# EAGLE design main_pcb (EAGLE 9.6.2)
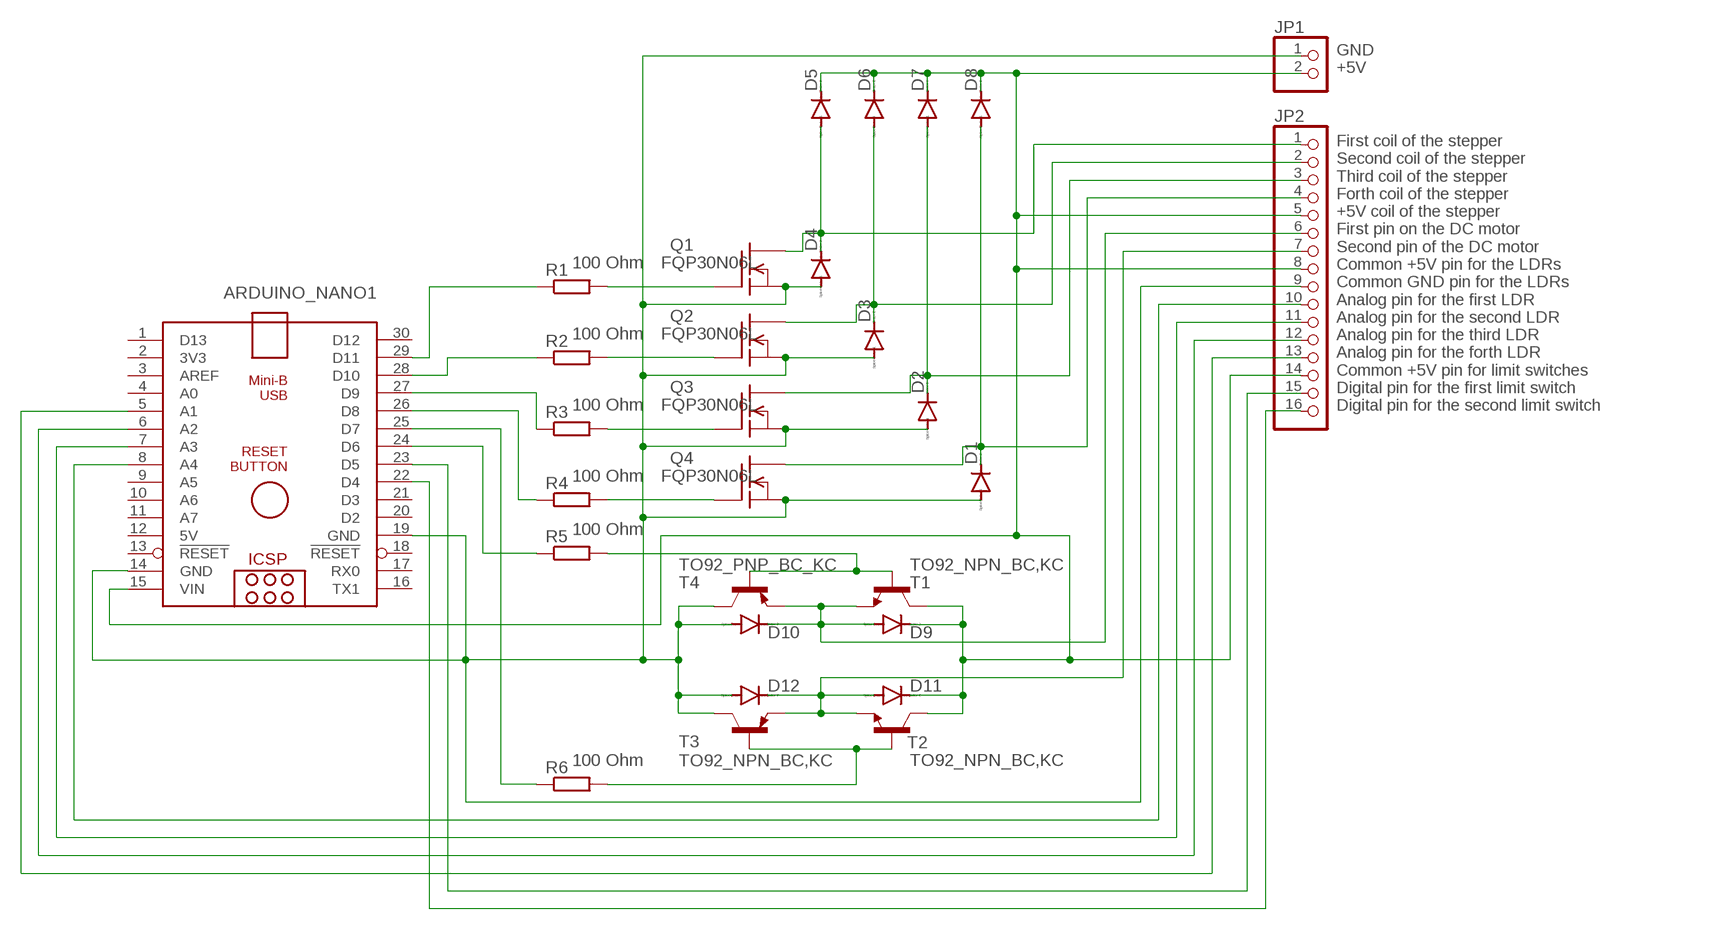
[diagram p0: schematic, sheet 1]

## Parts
ARDUINO_NANO1  ARDUINO_NANO  [ARDUINO_NANO]
D1  DIODY_1N,KADO35-7  [DO35-7]
D2  DIODY_1N,KADO35-7  [DO35-7]
D3  DIODY_1N,KADO35-7  [DO35-7]
D4  DIODY_1N,KADO35-7  [DO35-7]
D5  DIODY_1N,KADO35-7  [DO35-7]
D6  DIODY_1N,KADO35-7  [DO35-7]
D7  DIODY_1N,KADO35-7  [DO35-7]
D8  DIODY_1N,KADO35-7  [DO35-7]
D9  DIODY_1N,KADO35-7  [DO35-7]
D10  DIODY_1N,KADO35-7  [DO35-7]
D11  DIODY_1N,KADO35-7  [DO35-7]
D12  DIODY_1N,KADO35-7  [DO35-7]
JP1  PINHD-1X2  [1X02]
JP2  PINHD-1X16  [1X16]
Q1  BUZ10  [TO220]
Q2  BUZ10  [TO220]
Q3  BUZ10  [TO220]
Q4  BUZ10  [TO220]
R1  R-EU_0204/7  [0204/7]
R2  R-EU_0204/7  [0204/7]
R3  R-EU_0204/7  [0204/7]
R4  R-EU_0204/7  [0204/7]
R5  R-EU_0204/7  [0204/7]
R6  R-EU_0204/7  [0204/7]
T1  TO92_NPN_BC,KC  [TO92]
T2  TO92_NPN_BC,KC  [TO92]
T3  TO92_PNP_BC_KC  [TO92]
T4  TO92_PNP_BC_KC  [TO92]

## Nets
+5V: ARDUINO_NANO1.15(VIN) D5.C D6.C D7.C D8.C D9.C D11.C JP1.2 JP2.5 JP2.8 JP2.14 T1.3(C) T2.3(C)
GND: ARDUINO_NANO1.14(GND) ARDUINO_NANO1.19(GND) D1.A D2.A D3.A D4.A D10.A D12.A JP1.1 JP2.9 Q1.3(S) Q2.3(S) Q3.3(S) Q4.3(S) T3.3(C) T4.3(C)
N$1: ARDUINO_NANO1.29(D11) R1.1
N$2: ARDUINO_NANO1.28(D10) R2.1
N$3: ARDUINO_NANO1.27(D9) R3.1
N$4: ARDUINO_NANO1.26(D8) R4.1
N$5: Q1.1(G) R1.2
N$6: Q2.1(G) R2.2
N$7: Q3.1(G) R3.2
N$8: Q4.1(G) R4.2
N$9: D9.A D10.C JP2.6 T1.1(E) T4.1(E)
N$10: ARDUINO_NANO1.23(D5) JP2.15
N$11: ARDUINO_NANO1.22(D4) JP2.16
N$13: D11.A D12.C JP2.7 T2.1(E) T3.1(E)
N$14: D2.C D7.A JP2.3 Q3.2(D)
N$15: D3.C D6.A JP2.2 Q2.2(D)
N$16: D4.C D5.A JP2.1 Q1.2(D)
N$17: R5.2 T1.2(B) T4.2(B)
N$18: D1.C D8.A JP2.4 Q4.2(D)
N$19: R6.2 T2.2(B) T3.2(B)
N$20: ARDUINO_NANO1.25(D7) R6.1
N$21: ARDUINO_NANO1.24(D6) R5.1
N$23: ARDUINO_NANO1.8(A4) JP2.10
N$25: ARDUINO_NANO1.7(A3) JP2.11
N$26: ARDUINO_NANO1.6(A2) JP2.12
N$27: ARDUINO_NANO1.5(A1) JP2.13
Unconnected: ARDUINO_NANO1.1(D13) ARDUINO_NANO1.2(3V3) ARDUINO_NANO1.3(AREF) ARDUINO_NANO1.4(A0) ARDUINO_NANO1.9(A5) ARDUINO_NANO1.10(A6) ARDUINO_NANO1.11(A7) ARDUINO_NANO1.13(!RESET) ARDUINO_NANO1.16(TX1) ARDUINO_NANO1.17(RX0) ARDUINO_NANO1.18(!RESET) ARDUINO_NANO1.20(D2) ARDUINO_NANO1.21(D3) ARDUINO_NANO1.30(D12)

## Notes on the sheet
- GND
  +5V
- 100 Ohm | FQP30N06L
- 100 Ohm | FQP30N06L
- 100 Ohm | FQP30N06L
- First coil of the stepper
  Second coil of the stepper
  Third coil of the stepper
  Forth coil of the stepper
  +5V coil of the stepper
  First pin on the DC motor
  Second pin of the DC motor
  Common +5V pin for the LDRs
  Common GND pin for the LDRs
  Analog pin for the first LDR
  Analog pin for the second LDR
  Analog pin for the third LDR
  Analog pin for the forth LDR
  Common +5V pin for limit switches
  Digital pin for the first limit switch
  Digital pin for the second limit switch
- 100 Ohm | FQP30N06L
- 100 Ohm
- T4
- 100 Ohm
- T3
  TO92_NPN_BC,KC
- TO92_NPN_BC,KC

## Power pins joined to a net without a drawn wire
5V: ARDUINO_NANO1.12(5V)

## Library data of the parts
ARDUINO_NANO1 = ArduinoNanoV30:ARDUINO_NANO: Arduino Nano V3.0 Overview: The Arduino Nano is a small, complete, and breadboard-friendly board based on the ATmega328 (Arduino Nano 3.x) or ATmega168 (Arduino Nano 2.x). It has more or less the same functionality of the Arduino Duemilanove, but in a different package. It lacks only a DC power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
D1-D12 = knihovna praxe 123:DIODY_1N,KA: DIODE
JP1 = pinhead:PINHD-1X2: PIN HEADER
JP2 = pinhead:PINHD-1X16: PIN HEADER
Q1-Q4 = transistor-fet:BUZ10: N-Channel Enhancement MOSFET 50V; 20A; 0,080Ohm
R1-R6 = rcl:R-EU_: RESISTOR, European symbol; SPICEPREFIX: R
T1 T2 = knihovna praxe 123:TO92_NPN_BC,KC: NPN TRANSISTOR
T3 T4 = knihovna praxe 123:TO92_PNP_BC_KC: PNP Transistor

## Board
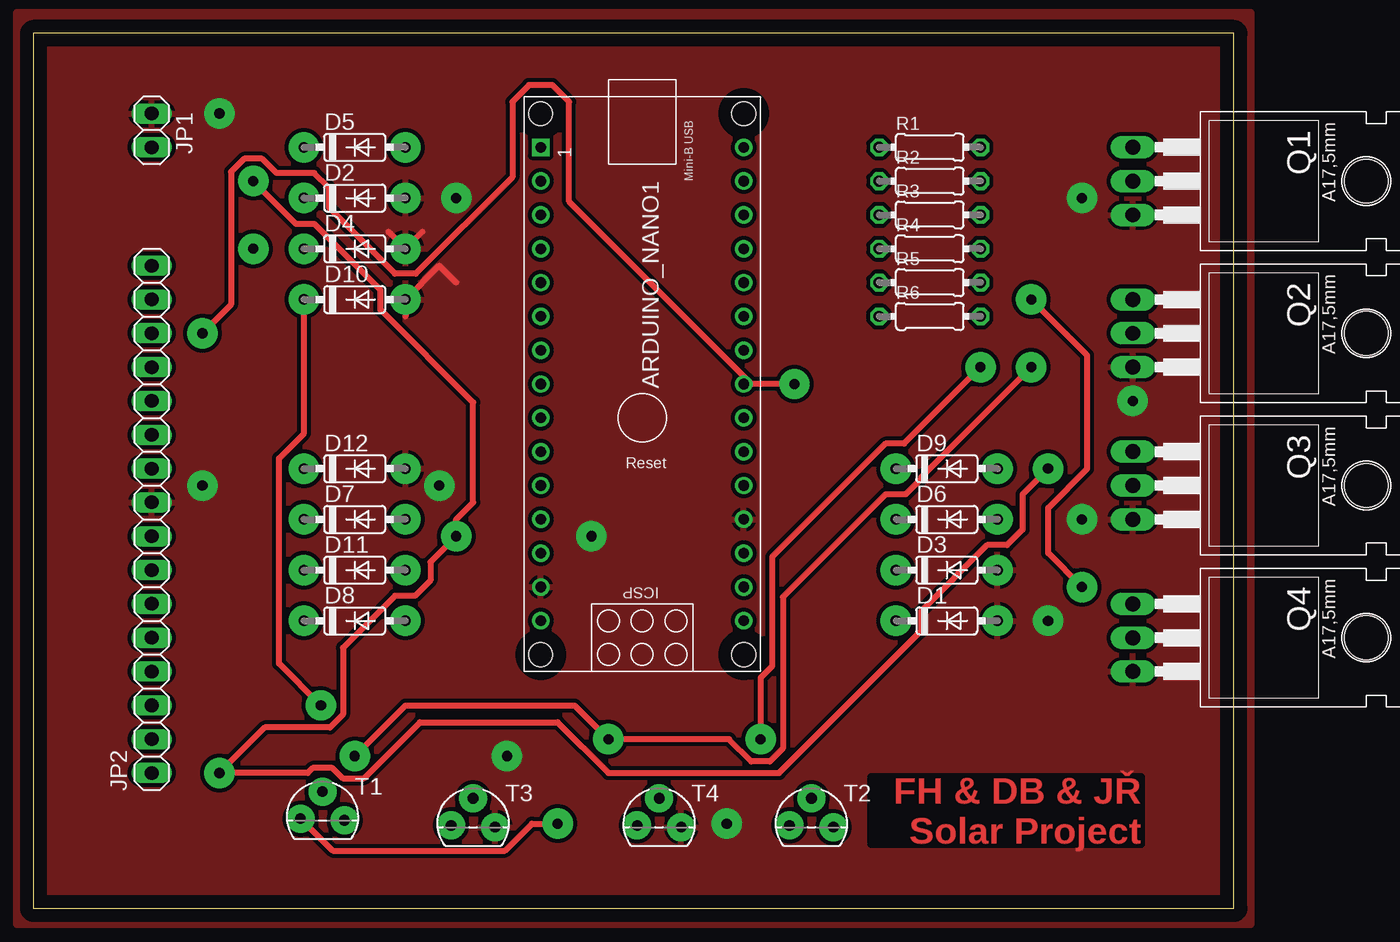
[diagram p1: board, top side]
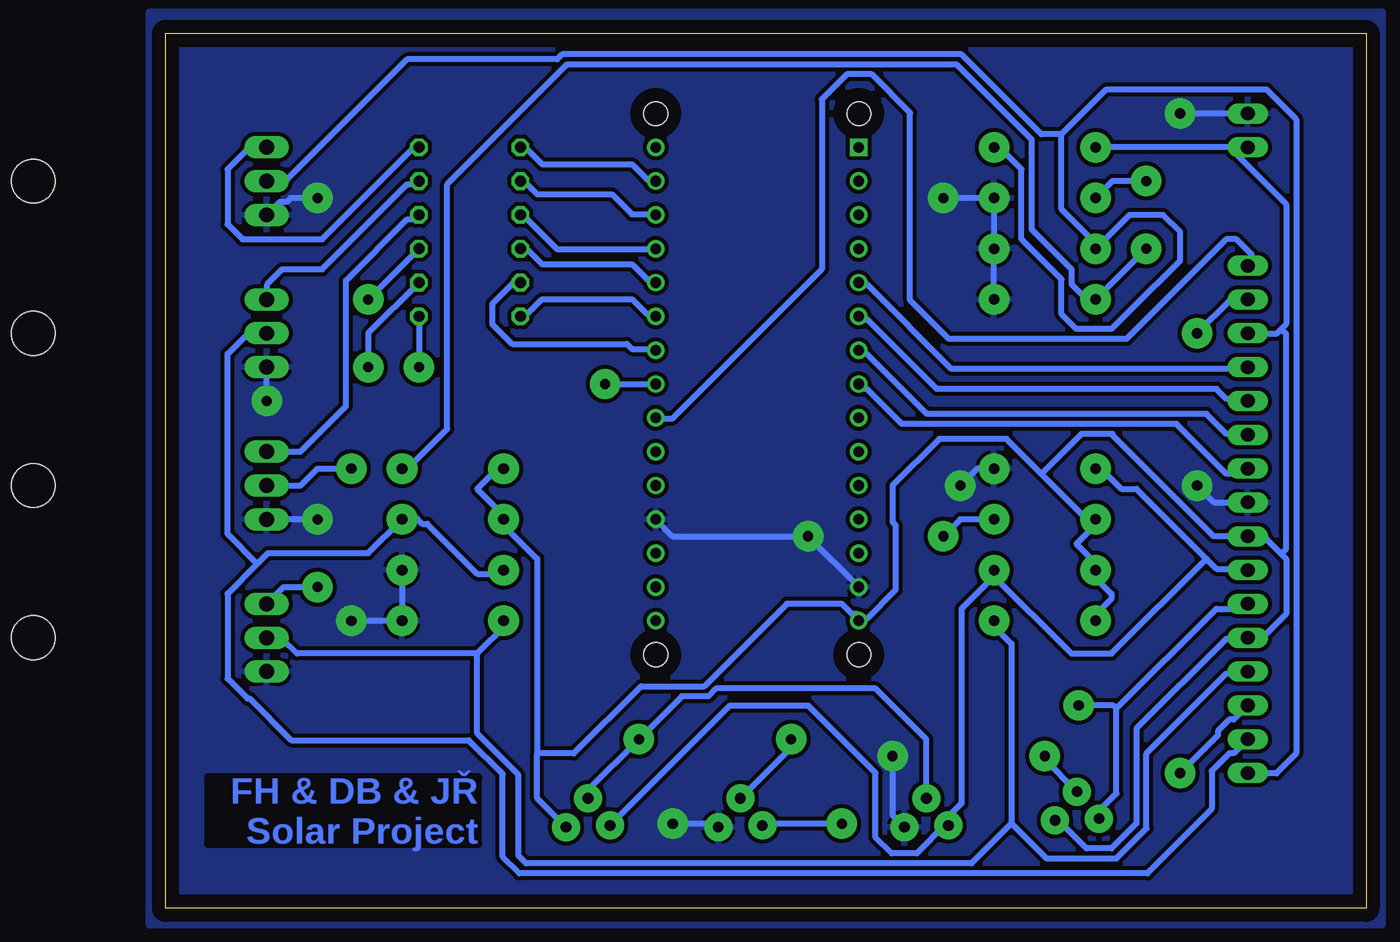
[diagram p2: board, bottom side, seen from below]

Size 90.15 x 65.71 mm. Coordinates in mm from the lower left corner, seen from the top.
Outline: 0,0 90.15,0 90.15,65.71 0,65.71 0,0
Copper layers (1*16): Top 0.035mm / dielectric 1.5mm / Bottom 0.035mm
Design rules "default *": minimum track width 0.45mm, minimum drill 0.35mm, track to track 0.3mm, track to pad 0.4mm, pad to pad 0.5mm, via to via 0.3mm, smd to smd 6mil, copper to edge 40mil, drill to drill 6mil, minimum pad ring 10mil, minimum via ring 8mil, stop-mask expansion 4mil, vias tented up to drill 0mil, thermal gap 10mil

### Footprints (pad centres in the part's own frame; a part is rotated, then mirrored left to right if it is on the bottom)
ARDUINO_NANO = drill 0.8 square: 1 -20.32,-7.62 | drill 0.8: 2 -17.78,-7.62; 3 -15.24,-7.62; 4 -12.7,-7.62; 5 -10.16,-7.62; 6 -7.62,-7.62; 7 -5.08,-7.62; 8 -2.54,-7.62; 9 0,-7.62; 10 2.54,-7.62; 11 5.08,-7.62; 12 7.62,-7.62; 13 10.16,-7.62; 14 12.7,-7.62; 15 15.24,-7.62; 16 15.24,7.62; 17 12.7,7.62; 18 10.16,7.62; 19 7.62,7.62; 20 5.08,7.62; 21 2.54,7.62; 22 0,7.62; 23 -2.54,7.62; 24 -5.08,7.62; 25 -7.62,7.62; 26 -10.16,7.62; 27 -12.7,7.62; 28 -15.24,7.62; 29 -17.78,7.62; 30 -20.32,7.62 | hole 1.778: -22.86,-7.62; -22.86,7.62; 17.78,7.62; 17.78,-7.62
DO35-7 = drill 0.8 pad 2.3: A 3.81,0; C -3.81,0
1X02 = drill 1.016 long: 1 -1.27,0; 2 1.27,0
1X16 = drill 1.016 long: 1 -19.05,0; 2 -16.51,0; 3 -13.97,0; 4 -11.43,0; 5 -8.89,0; 6 -6.35,0; 7 -3.81,0; 8 -1.27,0; 9 1.27,0; 10 3.81,0; 11 6.35,0; 12 8.89,0; 13 11.43,0; 14 13.97,0; 15 16.51,0; 16 19.05,0
TO220 = drill 1.118 long: 1 -2.54,-6.35; 2 0,-6.35; 3 2.54,-6.35 | hole 3.302: 0,11.176
0204/7 = drill 0.813 octagon: 1 -3.81,0; 2 3.81,0
TO92 = drill 0.8 pad 2.1: 1 -1.651,-0.127; 2 0,1.905; 3 1.651,-0.254

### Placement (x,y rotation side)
ARDUINO_NANO1  45.72,36.83 270 top
D1  68.58,21.59 0 top
D2  24.13,53.34 0 top
D3  68.58,25.4 0 top
D4  24.13,49.53 0 top
D5  24.13,57.15 0 top
D6  68.58,29.21 0 top
D7  24.13,29.21 0 top
D8  24.13,21.59 0 top
D9  68.58,33.02 0 top
D10  24.13,45.72 0 top
D11  24.13,25.4 0 top
D12  24.13,33.02 0 top
JP1  8.89,58.42 270 top
JP2  8.89,29.21 90 top
Q1  88.9,54.61 270 top
Q2  88.9,43.18 270 top
Q3  88.9,31.75 270 top
Q4  88.9,20.32 270 top
R1  67.31,57.15 0 top
R2  67.31,54.61 0 top
R3  67.31,52.07 0 top
R4  67.31,49.53 0 top
R5  67.31,46.99 0 top
R6  67.31,44.45 0 top
T1  21.72,6.86 0 top
T2  58.42,6.35 0 top
T3  33.02,6.35 0 top
T4  46.99,6.35 0 top

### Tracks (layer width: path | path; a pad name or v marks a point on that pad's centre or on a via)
+5V
  Bottom 0.45: 62.25,11.62 62.25,26.25 64.88,28.88 D6.C 64.5,29.25 66.75,31.5 65.25,33 64.88,33 D9.C | D8.C 20.25,21.75 20.25,22.12 19.12,23.25 19.12,23.62 20.62,25.12 D11.C 20.62,25.5 20.62,26.25 21.75,27.38 20.25,28.88 D7.C 20.62,28.88 24.38,32.62 | 37.88,21.75 37.5,21.75 35.34,23.91 35.34,28.79 35.56,29 35.56,31.75 32.06,35.25 27,35.25 24.38,32.62 | 6.38,43.5 6,43.88 6,52.88 9.38,56.25 | 6.38,43.5 6.75,43.12 8.62,43.12 JP2.14 | 9.38,56.25 9.38,56.62 9,57 JP1.2 | 19.88,57 20.25,57 D5.C 10.28,57.15 9.38,56.25 | 6.38,26.62 7.5,27.75 8.62,27.75 JP2.8 11.43,27.94 19.05,35.56 19.05,35.62 21.38,35.62 24.38,32.62 | 6.38,26.62 6,26.25 6,22.12 7.5,20.62 8.62,20.62 JP2.5 9,20.25 10.5,20.25 17.25,13.5 17.25,6.38 19.12,4.5 21,4.5 22.88,6.38 23.25,6.38 T1.3 | 6.38,43.5 6,43.12 6,27 6.38,26.62 | 37.88,21.75 38.25,22.12 38.62,22.12 39.38,22.88 43.5,22.88 49.7,16.68 54.44,16.68 59.49,11.62 62.25,11.62 | 37.88,21.75 ARDUINO_NANO1.15 | T2.3 62.25,8.28 62.25,11.62
GND  (via drill 0.76 pad 2.29)
  Top 0.45: 27.94,44.45 D10.A 30.48,48.26 31.75,46.99 | 29.21,50.8 D4.A 26.67,50.8
  Bottom 0.45: v35.56,11.43 35.56,6.99 T3.3 | T4.3 48.9,6.35 v52.07,6.35 | D12.A 29.21,33.02 v30.48,31.75 | v12.7,31.75 11.43,30.48 JP2.9 | JP1.1 v13.97,59.69 | v31.75,53.34 D2.A D4.A D10.A | ARDUINO_NANO1.14 v41.91,27.94 52.07,27.94 ARDUINO_NANO1.19 | D3.A D1.A v76.2,21.59 | v78.74,29.21 Q3.3 | v78.74,53.34 80.77,53.34 81.06,53.05 81.57,53.05 Q1.3 | v82.55,38.1 Q2.3
  pour Bottom: 0,67.31 91.44,67.31 91.44,-1.27 -1.27,-1.27 -1.27,67.31
  pour Top: -1.27,67.31 91.44,67.31 91.44,-1.27 -1.27,-1.27
N$1
  Bottom 0.45: ARDUINO_NANO1.29 53.62,54.75 54,54.75 55.12,55.88 61.88,55.88 63.38,57.38 R1.1
N$2
  Bottom 0.45: ARDUINO_NANO1.28 53.62,52.12 55.12,52.12 56.62,53.62 62.25,53.62 63.38,54.75 R2.1
N$3
  Bottom 0.45: ARDUINO_NANO1.27 53.62,49.5 60.75,49.5 63.38,52.12 R3.1
N$4
  Bottom 0.45: ARDUINO_NANO1.26 53.62,47.25 54,47.25 55.12,48.38 61.88,48.38 63.38,49.88 R4.1
N$5
  Bottom 0.45: R1.2 71.25,57 71.62,57 78.38,50.25 84.38,50.25 85.5,51.38 85.5,55.5 84,57 82.88,57 Q1.1
N$6
  Bottom 0.45: R2.2 71.25,54.38 72,54.38 78.38,48 81.38,48 82.5,46.88 82.5,45.75 Q2.1
N$7
  Bottom 0.45: R3.2 71.25,51.75 72,51.75 76.6,47.15 76.6,37.7 80.01,34.29 Q3.1
N$8  (via drill 0.76 pad 2.29)
  Top 0.45: v74.93,45.72 79.14,41.51 79.14,33.02 76.2,30.08 76.2,26.67 v78.74,24.13
  Bottom 0.45: Q4.1 81.28,24.13 v78.74,24.13 | R4.2 v74.93,45.72
N$9  (via drill 0.76 pad 2.29)
  Top 0.45: D10.C 20.32,35.67 18.45,33.8 18.45,18.39 v21.59,15.24 | v39.37,6.35 37.44,6.35 35.41,4.32 22.48,4.32 T1.1
  Bottom 0.45: 18.75,15 11.25,22.5 9,22.5 JP2.6 | 18.75,15 18.75,8.62 19.88,7.5 19.88,6.75 T1.1 | 20.62,45.75 21,45.75 22.12,46.88 22.12,48 25.12,51 25.12,57.75 30.75,63.38 60,63.38 69,54.38 69,36 71.62,33.38 72.38,33.38 D9.A | 20.62,45.75 D10.C | v16.51,49.53 20.29,45.75 20.62,45.75 | 18.75,15 18.99,15.24 v21.59,15.24 | v39.37,6.35 45.21,6.35 T4.1
N$10  (via drill 0.76 pad 2.29)
  Top 0.45: v57.15,39.37 53.93,39.37 40.23,53.07 40.23,60.57 38.98,61.82 37.22,61.82 35.97,60.57 35.97,54.91 28.72,47.66 27.16,47.66 22.2,52.62 22.2,54.12 21.1,55.22 18.26,55.22 17.2,56.28 15.82,56.28 14.84,55.3 14.84,45.32 v12.7,43.18
  Bottom 0.45: JP2.15 10.16,45.72 v12.7,43.18 | v57.15,39.37 ARDUINO_NANO1.23
N$11
  Bottom 0.45: ARDUINO_NANO1.22 53.25,36.75 52.12,36.75 40.88,48 40.88,60.75 39,62.62 37.12,62.62 34.24,59.74 34.24,45.67 31.32,42.75 18,42.75 10.5,50.25 9.75,50.25 8.62,49.12 8.62,48.38 JP2.16
N$13
  Bottom 0.45: 12,26.25 17.25,31.5 18.38,31.5 20.25,33.38 D12.C | 12,26.25 11.25,25.5 9,25.5 JP2.7 | 12,26.25 19.12,19.12 22.12,19.12 28.12,25.12 D11.A 27.75,25.12 30.38,22.5 30.38,7.88 31.12,7.12 31.12,6.38 T3.1 31.5,6.38 33.75,4.12 35.62,4.12 36.83,5.33 36.83,10.16 41.91,15.24 47.75,15.24 T2.1
N$14  (via drill 0.76 pad 2.29)
  Top 0.45: v16.51,54.61 19.71,51.41 21.1,51.41 26.07,46.44 26.07,44.94 33.02,37.99 33.02,30.48 31.75,29.21 v31.75,27.94 29.82,26 29.82,24.62 28.66,23.46 27.16,23.46 23.26,19.56 23.26,14.55 22.28,13.57 17.38,13.57 v13.97,10.16 20.6,10.16 20.98,10.54 22.45,10.54 23.23,9.76 24.82,9.76 29.03,13.97 39.37,13.97 43.18,10.16 55.99,10.16 66.64,20.81 66.64,22.31 71.61,27.27 73.11,27.27 74.27,28.43 74.27,31.09 v76.2,33.02
  Bottom 0.45: JP2.3 9.94,14.19 10.27,14.19 11.14,13.32 11.14,12.99 v13.97,10.16 | D7.A 30.48,29.21 v31.75,27.94 | v16.51,54.61 19.05,54.61 D2.C | Q3.2 80.01,31.75 78.74,33.02 v76.2,33.02
N$15
  Bottom 0.45: 83.25,25.88 85.5,23.62 85.5,17.25 84,15.75 83.82,15.75 80.7,12.63 67.38,12.63 64.84,10.09 64.84,3.88 63.59,2.62 16.43,2.62 11.59,7.46 11.59,10.32 10.27,11.65 9.94,11.65 JP2.2 | 72.75,29.25 D6.A | 83.25,25.88 85.5,28.12 85.5,41.62 84,43.12 82.88,43.12 Q2.2 | D3.C 64.88,25.12 66.75,25.12 70.5,28.88 70.88,28.88 71.25,29.25 72.38,29.25 D6.A | 83.25,25.88 82.45,26.67 74.93,26.67 D6.A
N$16
  Bottom 0.45: 22.88,58.12 19.5,61.5 7.5,61.5 5.25,59.25 5.25,11.62 6.75,10.12 8.62,10.12 JP2.1 | 22.88,58.12 22.88,52.5 20.25,49.88 D4.C 20.62,49.5 20.49,49.36 17.78,52.07 15.24,52.07 13.97,50.8 13.97,48.66 17.62,45 19.12,43.5 21.75,43.5 22.88,44.62 22.88,47.25 25.88,50.25 25.88,55.5 27.38,57 27.75,57 D5.A | 22.88,58.12 24.38,58.12 30.38,64.12 60.38,64.12 60.75,63.75 72,63.75 81,54.75 82.5,54.75 Q1.2
N$17  (via drill 0.76 pad 2.29)
  Top 0.45: v74.93,40.64 66.64,32.35 66.64,32.24 65.49,31.09 63.99,31.09 56.28,23.37 56.28,12.01 55.3,11.03 53.92,11.03 52.25,12.7 v43.18,12.7 40.64,15.24 27.94,15.24 v24.13,11.43
  Bottom 0.45: T4.2 43.18,12.06 v43.18,12.7 | T1.2 24.13,11.18 v24.13,11.43 | R5.2 74.93,43.18 v74.93,40.64
N$18
  Bottom 0.45: 66.75,19.12 80.25,19.12 81.38,20.25 82.5,20.25 Q4.2 | 66.75,19.12 64.5,21.38 D1.C | 26.62,6.38 24,3.75 18.75,3.75 16.5,6 16.5,11.62 10.5,17.62 9,17.62 JP2.4 | 26.62,6.38 26.62,19.88 28.12,21.38 D8.A | 66.75,19.12 66.75,13.12 63.64,10.02 63.64,3.95 63.06,3.38 29.62,3.38 26.62,6.38
N$19  (via drill 0.76 pad 2.29)
  Top 0.45: v71.12,40.64 65.38,34.9 63.99,34.9 55.47,26.37 55.47,18.17 54.61,17.31 v54.61,12.7
  Bottom 0.45: 58.19,8.62 T2.2 58.42,8.89 v54.61,12.7 51.38,15.93 49.39,15.93 48.8,16.51 36.83,16.51 33.02,12.7 T3.2 | R6.2 v71.12,40.64
N$20
  Bottom 0.45: ARDUINO_NANO1.25 53.62,44.62 54,44.62 55.12,45.75 61.88,45.75 63.38,44.25 R6.1
N$21
  Bottom 0.45: ARDUINO_NANO1.24 53.62,42 55.12,42 55.5,42.38 64.12,42.38 65.62,43.88 65.62,45.38 63.75,47.25 R5.1
N$23
  Bottom 0.45: ARDUINO_NANO1.8 37.88,39 37.5,39 34.88,36.38 14.25,36.38 10.5,32.62 9.38,32.62 9,33 JP2.10
N$25
  Bottom 0.45: ARDUINO_NANO1.7 37.88,41.62 37.5,41.62 33,37.12 12,37.12 10.5,35.62 9,35.62 JP2.11
N$26
  Bottom 0.45: ARDUINO_NANO1.6 37.88,44.25 37.5,44.25 32.25,39 11.25,39 10.5,38.25 9,38.25 JP2.12
N$27
  Bottom 0.45: ARDUINO_NANO1.5 37.88,46.88 37.5,46.88 31.12,40.5 9,40.5 JP2.13

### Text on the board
Top: FH & DB & JŘ / Solar Project
Bottom: FH & DB & JŘ / Solar Project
